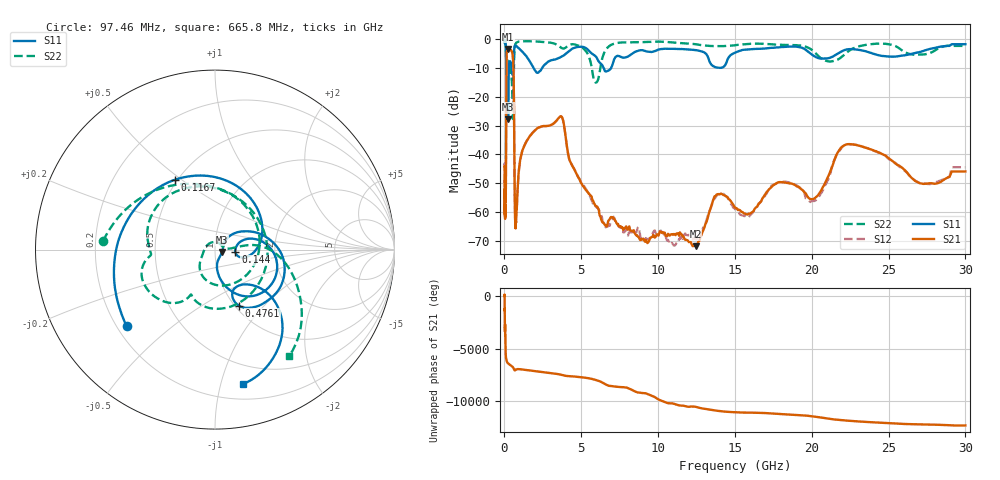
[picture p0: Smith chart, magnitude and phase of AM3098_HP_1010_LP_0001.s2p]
! Date/Time: Thu, Feb 28, 2019 8:41 AM
! Network Analyzer: Agilent Technologies E8364B Rev: A.07.50.67
! Sweep from 0.010 to 30.000 GHz, 1601 Points, Sweep Type: LOG
! Power Supply: 5.022 V, 0.002 A
# Hz S DB R 50
!freq MagS11 AngS11 MagS21 AngS21 MagS12 AngS12 MagS22 AngS22
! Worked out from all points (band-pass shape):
!   1601 points, 10 MHz to 30 GHz, reference 50 ohm
!   highest |S21| = -3.33 dB at 242.3 MHz (marker M1); lowest = -71.9 dB at 12.43 GHz (marker M2)
!   |S21| within 3 dB of the highest: 133.1 MHz to 551.2 MHz (418.1 MHz wide, 122 % of centre)
!   lowest |S11| = -27.7 dB at 238.7 MHz (marker M3), VSWR 1.09, Z = 54 - j1.49 ohm
!   |S11| at or under -10 dB: 199.4 MHz to 292.3 MHz (92.86 MHz wide, 37.8 % of centre); 1.898 GHz to 2.441 GHz (543.6 MHz wide, 25.1 % of centre); 6.465 GHz to 6.932 GHz (466.4 MHz wide, 6.96 % of centre)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
!   |S22| runs from -27.6 to -0.5 dB; largest |S21 - S12| = 0.0099
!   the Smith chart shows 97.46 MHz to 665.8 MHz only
!   S11 on the Smith chart (normalised r, x): 97.46 MHz: 0.24, -0.35; 116.7 MHz: 0.48, +0.47; 144 MHz: 1.26, -0.04; 476.1 MHz: 1.04, -0.74; 665.8 MHz: 0.33, -1.18
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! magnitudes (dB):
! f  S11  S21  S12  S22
! 10 MHz  -0.4  -44.0  -43.8  -0.5
! 38.04 MHz  -0.4  -59.0  -58.7  -0.8
! 97.46 MHz  -3.7  -46.4  -47.8  -4.1
! 116.7 MHz  -7.0  -17.9  -18.0  -10.6
! 144 MHz  -18.8  -4.8  -4.7  -10.9
! 144.7 MHz  -18.9  -4.7  -4.7  -10.8
! 191.5 MHz  -9.0  -3.8  -3.8  -7.2
! 238.7 MHz  -27.7  -3.3  -3.3  -8.9
! 242.3 MHz  -27.2  -3.3  -3.3  -8.9
! 476.1 MHz  -9.3  -4.1  -4.1  -14.0
! 550.5 MHz  -11.9  -6.3  -6.2  -27.3
! 605.4 MHz  -5.6  -15.6  -15.6  -11.6
! 665.8 MHz  -2.3  -53.2  -52.5  -2.8
! 735.8 MHz  -2.1  -64.2  -61.8  -1.3
! 1.034 GHz  -3.6  -41.6  -41.9  -0.7
! 2.084 GHz  -11.5  -31.1  -31.1  -0.7
! 3.704 GHz  -6.0  -26.8  -26.8  -2.9
! 5.959 GHz  -6.0  -57.9  -58.1  -15.0
! 7.926 GHz  -6.2  -65.0  -67.0  -1.0
! 12.43 GHz  -3.7  -71.9  -69.4  -1.6
! 22.56 GHz  -3.4  -36.4  -36.5  -3.5
! 30 GHz  -1.7  -45.9  -44.4  -2.2
